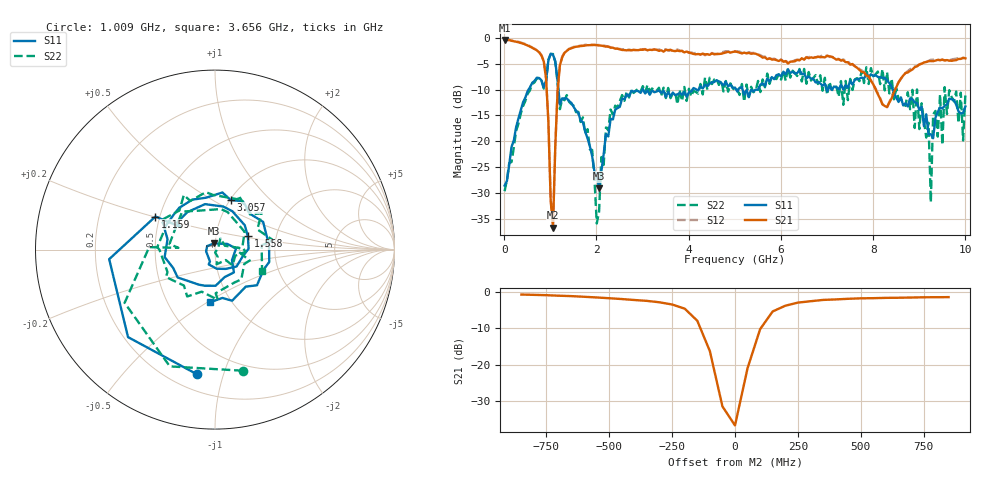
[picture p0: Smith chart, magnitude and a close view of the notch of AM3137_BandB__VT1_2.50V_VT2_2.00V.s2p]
! Date/Time: Tue, Nov 13, 2018 4:51 PM
! Network Analyzer: Agilent Technologies E8364B Rev: A.07.50.67
! Sweep from 0.010 to 10.000 GHz, 201 Points, Sweep Type: LIN
! Power Supply: 2.501 V, 0.001 A
# Hz S DB R 50
!freq MagS11 AngS11 MagS21 AngS21 MagS12 AngS12 MagS22 AngS22
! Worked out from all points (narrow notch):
!   201 points, 10 MHz to 10 GHz, reference 50 ohm
!   highest |S21| = -0.40 dB at 10 MHz (marker M1); lowest = -36.7 dB at 1.059 GHz (marker M2)
!   notch at M2: 33.4 dB deep, 142 MHz wide at half that depth
!   lowest |S11| = -29.1 dB at 2.058 GHz (marker M3), VSWR 1.07, Z = 49.4 + j3.44 ohm
!   |S11| at or under -10 dB: 1.177 GHz to 2.999 GHz (1.822 GHz wide, 87.3 % of centre); 3.014 GHz to 4.084 GHz (1.07 GHz wide, 30.1 % of centre); 8.424 GHz to end of sweep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
!   |S22| runs from -35.9 to -3.1 dB; largest |S21 - S12| = 0.036
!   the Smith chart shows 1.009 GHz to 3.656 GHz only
!   S11 on the Smith chart (normalised r, x): 1.009 GHz: 0.30, -0.82; 1.159 GHz: 0.47, +0.20; 1.558 GHz: 1.43, +0.22; 3.057 GHz: 1.01, +0.61; 3.656 GHz: 0.80, -0.51
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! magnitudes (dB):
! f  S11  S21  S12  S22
! 10 MHz  -28.6  -0.4  -0.3  -29.6
! 859.2 MHz  -9.6  -4.6  -4.5  -9.8
! 1.009 GHz  -3.1  -31.4  -31.2  -3.2
! 1.059 GHz  -3.3  -36.7  -36.1  -3.1
! 1.159 GHz  -8.4  -10.2  -10.1  -8.7
! 1.558 GHz  -14.1  -1.7  -1.7  -14.4
! 1.708 GHz  -16.3  -1.6  -1.5  -15.4
! 2.058 GHz  -29.1  -1.5  -1.4  -33.6
! 2.308 GHz  -15.6  -1.9  -1.8  -13.9
! 3.057 GHz  -10.8  -2.2  -2.2  -10.6
! 3.357 GHz  -10.2  -2.5  -2.3  -9.7
! 3.656 GHz  -10.6  -2.5  -2.5  -10.8
! 5.005 GHz  -9.6  -2.7  -2.6  -10.3
! 6.703 GHz  -7.9  -3.9  -3.7  -7.8
! 8.352 GHz  -8.8  -12.5  -12.4  -10.8
! 8.951 GHz  -12.7  -5.5  -5.4  -10.0
! 9.201 GHz  -18.6  -4.5  -4.5  -16.4
! 9.251 GHz  -18.7  -4.5  -4.2  -31.8
! 9.301 GHz  -19.4  -4.5  -4.2  -14.8
! 9.9 GHz  -14.6  -4.1  -4.1  -10.6
! 9.95 GHz  -14.5  -3.9  -4.0  -19.8
! 10 GHz  -13.3  -4.0  -3.9  -10.9
